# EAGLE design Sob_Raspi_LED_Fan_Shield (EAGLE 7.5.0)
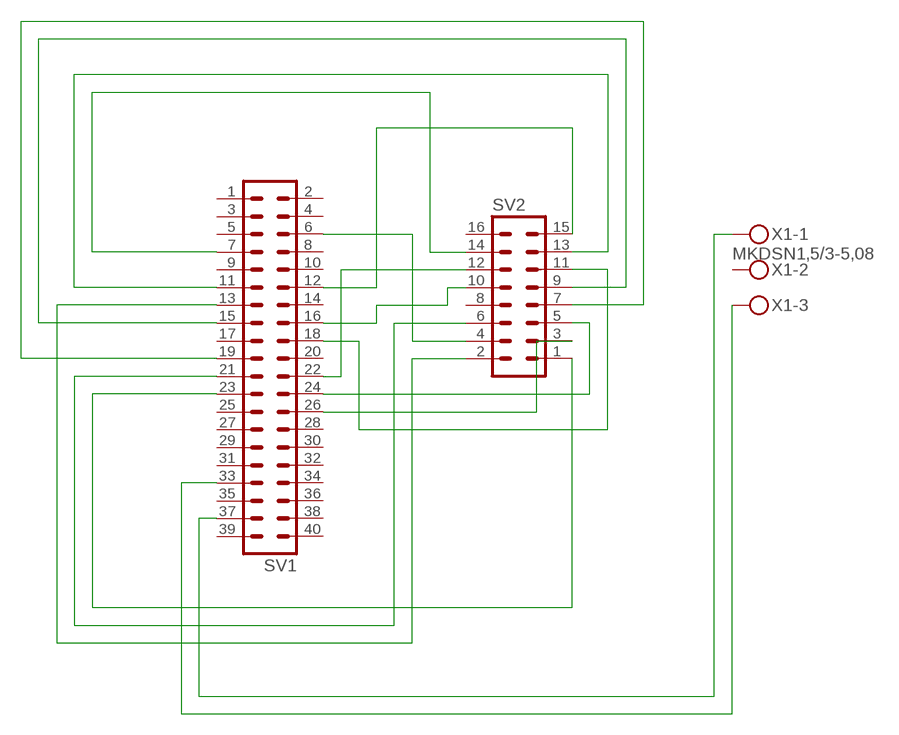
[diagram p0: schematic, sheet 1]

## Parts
SV1  MA20-2  [MA20-2]
SV2  ML16  [ML16]
X1  MKDSN1,5/3-5,08  [MKDSN1,5/3-5,08]

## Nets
N$1: SV1.7 SV2.14
N$2: SV1.11 SV2.13
N$3: SV1.13 SV2.2
N$4: SV1.15 SV2.9
N$5: SV1.19 SV2.7
N$6: SV1.21 SV2.6
N$7: SV1.23 SV2.1
N$8: SV1.33 X1.3
N$9: SV1.37 X1.1
N$10: SV1.12 SV2.15
N$11: SV1.16 SV2.10
N$12: SV1.18 SV2.11
N$13: SV1.22 SV2.12
N$14: SV1.24 SV2.5
N$15: SV1.26 SV2.3
N$16: SV1.6 SV2.4
Unconnected: SV1.1 SV1.2 SV1.3 SV1.4 SV1.5 SV1.8 SV1.9 SV1.10 SV1.14 SV1.17 SV1.20 SV1.25 SV1.27 SV1.28 SV1.29 SV1.30 SV1.31 SV1.32 SV1.34 SV1.35 SV1.36 SV1.38 SV1.39 SV1.40 SV2.8 SV2.16 X1.2

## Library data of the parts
SV1 = con-lstb:MA20-2: PIN HEADER; OC_FARNELL: unknown; OC_NEWARK: unknown
SV2 = con-harting-ml:ML16: HARTING; OC_FARNELL: unknown; OC_NEWARK: unknown
X1 = con-phoenix-508:MKDSN1,5/3-5,08: MKDSN 1,5/ 3-5,08 Printklemme Nennstrom: 13,5 A Nennspannung: 250 V Rastermaß: 5,08 mm Polzahl: 3 Anschlussart: Schraubanschluss Montage: Löten Anschlussrichtung Leiter/Platine: 0 ° Artikelnummer: 1729131 Source: http://eshop.phoenixcontact.com .. 1729131.pdf

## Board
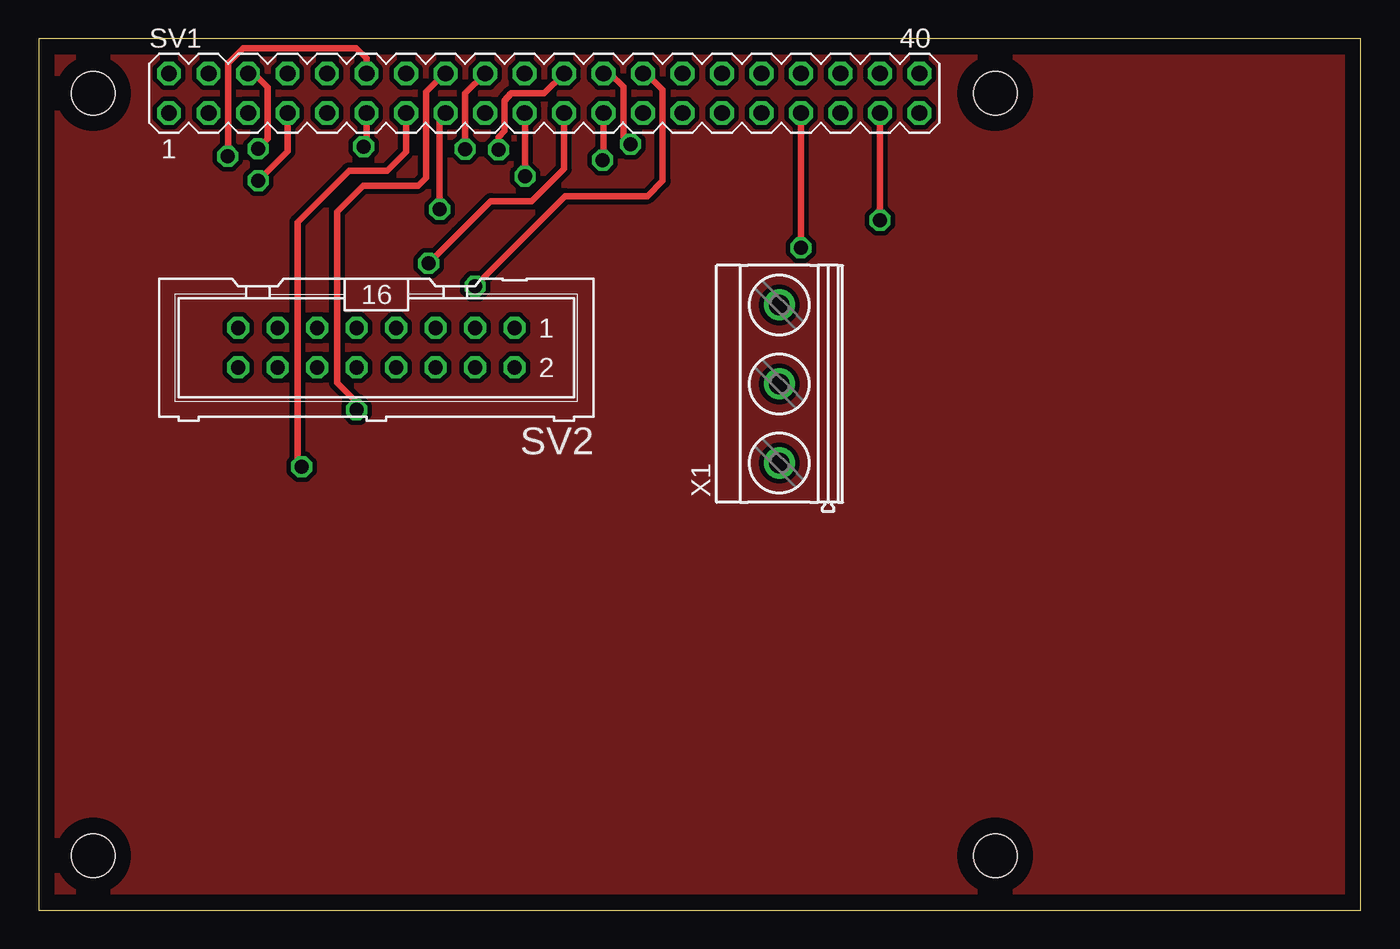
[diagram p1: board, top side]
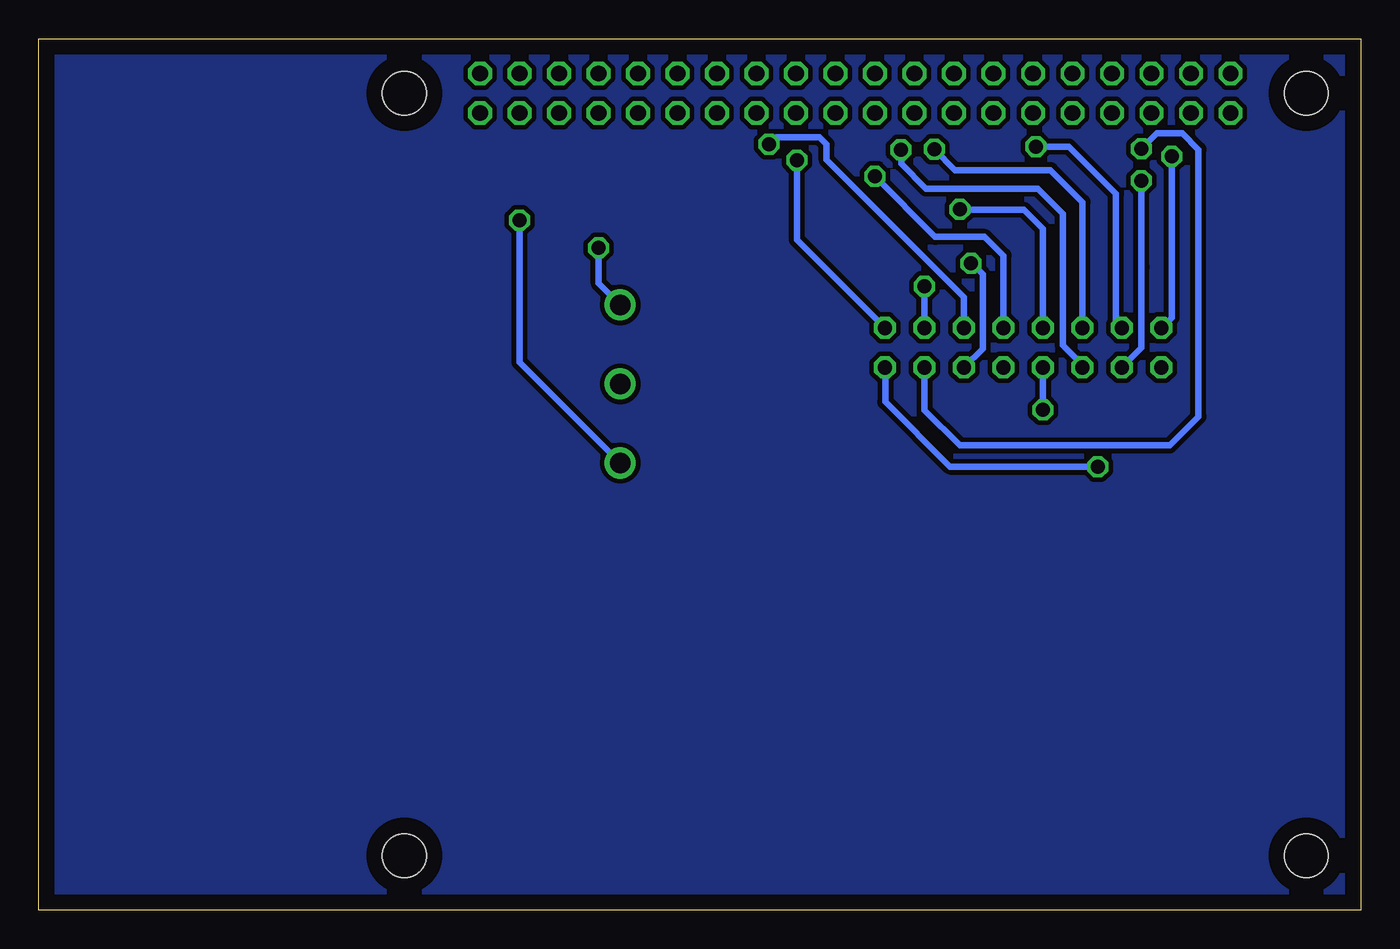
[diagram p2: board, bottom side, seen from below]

Size 85 x 56 mm. Coordinates in mm from the lower left corner, seen from the top.
Outline: 0,0 85,0 85,56 0,56 0,0
Copper layers (1*16): Top 0.035mm / dielectric 1.5mm / Bottom 0.035mm
Design rules "default *": minimum track width 10mil, minimum drill 24mil, track to track 12mil, track to pad 12mil, pad to pad 12mil, via to via 12mil, smd to smd 8mil, copper to edge 40mil, drill to drill 8mil, minimum pad ring 10mil, minimum via ring 8mil, stop-mask expansion 4mil, vias tented up to drill 0mil, thermal gap 10mil
Holes 2.8 mm at 3.5,52.5 61.5,52.5 61.5,3.5 3.5,3.5

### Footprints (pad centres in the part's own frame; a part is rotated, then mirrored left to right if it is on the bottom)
MA20-2 = drill 1.016 octagon: 1 -24.13,-1.27; 2 -24.13,1.27; 3 -21.59,-1.27; 4 -21.59,1.27; 5 -19.05,-1.27; 6 -19.05,1.27; 7 -16.51,-1.27; 8 -16.51,1.27; 9 -13.97,-1.27; 10 -13.97,1.27; 11 -11.43,-1.27; 12 -11.43,1.27; 13 -8.89,-1.27; 14 -8.89,1.27; 15 -6.35,-1.27; 16 -6.35,1.27; 17 -3.81,-1.27; 18 -3.81,1.27; 19 -1.27,-1.27; 20 -1.27,1.27; 21 1.27,-1.27; 22 1.27,1.27; 23 3.81,-1.27; 24 3.81,1.27; 25 6.35,-1.27; 26 6.35,1.27; 27 8.89,-1.27; 28 8.89,1.27; 29 11.43,-1.27; 30 11.43,1.27; 31 13.97,-1.27; 32 13.97,1.27; 33 16.51,-1.27; 34 16.51,1.27; 35 19.05,-1.27; 36 19.05,1.27; 37 21.59,-1.27; 38 21.59,1.27; 39 24.13,-1.27; 40 24.13,1.27
ML16 = drill 0.914 octagon: 1 -8.89,-1.27; 2 -8.89,1.27; 3 -6.35,-1.27; 4 -6.35,1.27; 5 -3.81,-1.27; 6 -3.81,1.27; 7 -1.27,-1.27; 8 -1.27,1.27; 9 1.27,-1.27; 10 1.27,1.27; 11 3.81,-1.27; 12 3.81,1.27; 13 6.35,-1.27; 14 6.35,1.27; 15 8.89,-1.27; 16 8.89,1.27
MKDSN1,5/3-5,08 = drill 1.3 pad 2: 1 -7.641,0.025; 2 -2.561,0.025; 3 2.519,0.025

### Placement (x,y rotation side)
SV1  32.5,52.5 0 top
SV2  21.7,36.15 180 top
X1  47.64,36.38 90 top

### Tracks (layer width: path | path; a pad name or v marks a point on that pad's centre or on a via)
GND
  pour Top: 0.09,56.28 85.63,56.28 85.63,0 0.09,0
  pour Bottom: 0.07,56.27 84.99,56.27 84.99,0.2 0.07,0.2
N$1  (via drill 0.9)
  Top 0.406: v14.11,46.89 15.99,48.77 SV1.7
  Bottom 0.406: SV2.14 14.1,36.13 14.1,41.35 14.11,41.36 v14.11,46.89
N$2  (via drill 0.9)
  Top 0.406: v20.89,49.08 21.07,49.26 SV1.11
  Bottom 0.406: SV2.13 15.73,37.8 15.73,46.04 18.77,49.08 v20.89,49.08
N$3  (via drill 0.9)
  Top 0.406: v16.91,28.5 16.64,28.77 16.64,44.22 19.95,47.53 22.39,47.53 23.61,48.75 SV1.13
  Bottom 0.406: SV2.2 30.57,34.86 30.57,32.67 26.4,28.5 v16.91,28.5
N$4  (via drill 0.9)
  Top 0.406: v25.78,45.04 25.78,50.86 SV1.15
  Bottom 0.406: SV2.9 20.43,43.79 21.65,45.01 25.75,45.01 v25.78,45.04
N$5  (via drill 0.9)
  Top 0.406: v31.25,47.16 31.25,51.21 SV1.19
  Bottom 0.406: SV2.7 22.97,42.07 24.18,43.28 27.37,43.28 v31.25,47.16
N$6  (via drill 0.9)
  Top 0.406: v25.05,41.57 29.05,45.57 31.69,45.57 33.77,47.65 SV1.21
  Bottom 0.406: SV2.6 24.3,36.09 24.3,40.86 25.01,41.57 v25.05,41.57
N$7  (via drill 0.9)
  Top 0.406: v36.26,48.21 36.31,48.26 SV1.23
  Bottom 0.406: SV2.1 36.26,43.09 v36.26,48.21
N$8  (via drill 0.9)
  Top 0.406: v49,42.56 v49.01,42.57 SV1.33
  Bottom 0.406: X1.3 49,40.28 v49,42.56
N$9  (via drill 0.9)
  Top 0.406: v54.1,44.34 v54.09,44.35 SV1.37
  Bottom 0.406: X1.1 54.1,35.22 v54.1,44.34
N$10  (via drill 0.9)
  Top 0.406: v12.15,48.44 12.18,48.47 12.18,54.44 13.15,55.41 20.41,55.41 21.07,54.75 SV1.12
  Bottom 0.406: SV2.15 12.15,38.08 v12.15,48.44
N$11  (via drill 0.9)
  Top 0.406: v20.42,32.15 20.42,32.65 19.17,33.9 19.17,44.88 20.86,46.57 24.38,46.57 24.89,47.08 24.89,52.59 26.07,53.77 SV1.16
  Bottom 0.406: SV2.10 v20.43,32.16 v20.42,32.15
N$12  (via drill 0.9)
  Top 0.406: v27.42,48.92 27.42,52.52 SV1.18
  Bottom 0.406: SV2.11 17.89,45.5 19.95,47.56 26.08,47.56 v27.42,48.92
N$13  (via drill 0.9)
  Top 0.406: v29.56,48.87 29.56,49.68 29.96,50.08 29.96,52.03 30.37,52.5 32.48,52.5 SV1.22
  Bottom 0.406: SV2.12 17.89,35.06 19.15,36.32 19.15,44.76 20.77,46.38 27.94,46.38 29.52,47.96 29.52,48.83 v29.56,48.87
N$14  (via drill 0.9)
  Top 0.406: v38.05,49.24 37.59,49.7 37.59,52.92 36.74,53.77 SV1.24
  Bottom 0.406: SV2.5 25.51,39.39 34.34,48.22 34.34,49.22 34.81,49.69 37.6,49.69 v38.05,49.24
N$15  (via drill 0.9)
  Top 0.406: v28.05,40.09 33.85,45.89 39.13,45.89 40.12,46.88 40.12,52.73 39.08,53.77 SV1.26
  Bottom 0.406: SV2.3 v28.05,40.09
N$16  (via drill 0.9)
  Top 0.406: v14.09,48.94 14.72,49.57 14.72,52.89 13.84,53.77 SV1.6
  Bottom 0.406: SV2.4 28.05,32.14 25.78,29.87 12.27,29.87 10.43,31.71 10.43,48.88 11.48,49.93 13.1,49.93 v14.09,48.94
